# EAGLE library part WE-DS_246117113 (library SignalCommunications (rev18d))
WE-DS D-SUB-Filter Connectors Bent 90° Characteristics Standard type filtered with 1000 pF High attenuation of more than 40 dB @ 180 MHz Low size: 6.3 mm Rated voltage: 125 VDC Rated current @ 20 ºC: 5 A Withstand voltage: 250 VRMS Insulation resistance: min. 1000 MΩ Operating temperature: –55 ºC to +125 ºC Applications Filtering of interfaces External connection to -printer -sensor -display Details see: http://katalog.we-online.de/en/pbs/D-SUB-Filter Bent 90° Created on 2015-05-04 2015 (C) Wurth Elektronik
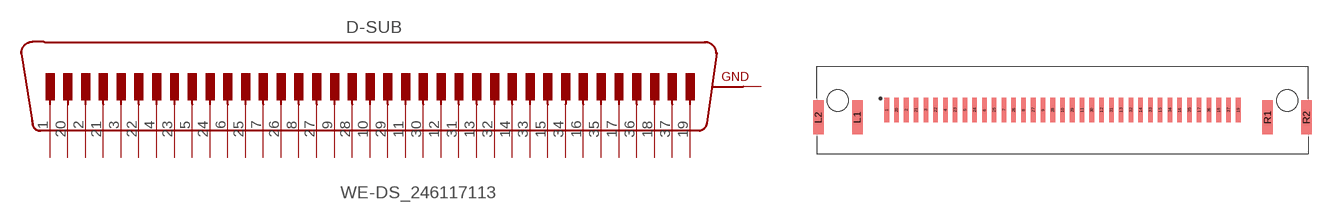
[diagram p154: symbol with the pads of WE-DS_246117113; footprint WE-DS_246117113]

Designator prefix D-SUB

## WE-DS_246117113 (WE-NUMBER: 246117113/37Pins_male)  [WE-DS_246117113]
1  1  pas
2  2  pas
3  3  pas
4  4  pas
5  5  pas
6  6  pas
7  7  pas
8  8  pas
9  9  pas
10  10  pas
11  11  pas
12  12  pas
13  13  pas
14  14  pas
15  15  pas
16  16  pas
17  17  pas
18  18  pas
19  19  pas
20  20  pas
21  21  pas
22  22  pas
23  23  pas
24  24  pas
25  25  pas
26  26  pas
27  27  pas
28  28  pas
29  29  pas
30  30  pas
31  31  pas
32  32  pas
33  33  pas
34  34  pas
35  35  pas
36  36  pas
37  37  pas
L1  GND  pwr
L2  GND  pwr
R1  GND  pwr
R2  GND  pwr

## Footprint WE-DS_246117113 (pad centres in mm)
smd 0.65 x 3.5: 1 -24.84,0; 2 -22.08,0; 3 -19.32,0; 4 -16.56,0; 5 -13.8,0; 6 -11.04,0; 7 -8.28,0; 8 -5.52,0; 9 -2.76,0; 10 0,0; 11 2.76,0; 12 5.52,0; 13 8.28,0; 14 11.04,0; 15 13.8,0; 16 16.56,0; 17 19.32,0; 18 22.08,0; 19 24.84,0; 20 -23.46,0; 21 -20.7,0; 22 -17.94,0; 23 -15.18,0; 24 -12.42,0; 25 -9.66,0; 26 -6.9,0; 27 -4.14,0; 28 -1.38,0; 29 1.38,0; 30 4.14,0; 31 6.9,0; 32 9.66,0; 33 12.42,0; 34 15.18,0; 35 17.94,0; 36 20.7,0; 37 23.46,0
smd 1.5 x 4.8: L1 -29,-1.05; L2 -34.5,-1.05; R1 29,-1.05; R2 34.5,-1.05
hole 3 at -31.75,1.35
hole 3 at 31.75,1.35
